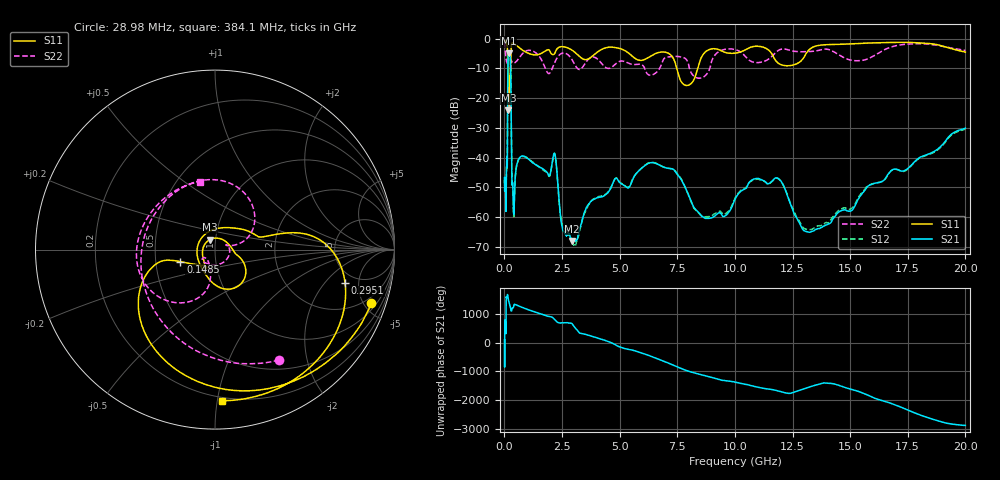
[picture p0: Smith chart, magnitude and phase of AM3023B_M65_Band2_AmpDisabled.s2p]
!Agilent Technologies,E8364B,MY43040894,A.07.50.67
!Agilent E8364B: A.07.50.67
!Date: Tuesday, October 27, 2020 10:48:38
!Correction: S11(Full 2 Port(1,2))
!S21(Full 2 Port(1,2))
!S12(Full 2 Port(1,2))
!S22(Full 2 Port(1,2))
!S2P File: Measurements: S11, S21, S12, S22:Log Frequency Sweep
# Hz S  dB  R 50
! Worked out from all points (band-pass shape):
!   3201 points, 10 MHz to 20 GHz, reference 50 ohm
!   highest |S21| = -4.86 dB at 193.4 MHz (marker M1); lowest = -68.0 dB at 2.92 GHz (marker M2)
!   |S21| within 3 dB of the highest: 154.6 MHz to 264.8 MHz (110.2 MHz wide, 52.6 % of centre)
!   lowest |S11| = -24.1 dB at 175.4 MHz (marker M3), VSWR 1.13, Z = 46.9 + j5.22 ohm
!   |S11| at or under -10 dB: 145.6 MHz to 264.5 MHz (118.9 MHz wide, 58 % of centre); 7.479 GHz to 8.387 GHz (907.2 MHz wide, 11.4 % of centre)
!   |S22| runs from -23.7 to -1.3 dB; largest |S21 - S12| = 0.0085
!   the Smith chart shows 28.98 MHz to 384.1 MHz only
!   S11 on the Smith chart (normalised r, x): 28.98 MHz: 1.43, -5.64; 148.5 MHz: 0.67, -0.09; 295.1 MHz: 3.96, -3.39; 384.1 MHz: 0.18, -1.03
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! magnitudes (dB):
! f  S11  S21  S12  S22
! 10 MHz  -0.6  -47.6  -47.6  -1.3
! 28.98 MHz  -0.7  -49.0  -48.9  -3.0
! 35.55 MHz  -0.8  -48.7  -48.4  -3.6
! 69.3 MHz  -1.1  -57.6  -56.0  -6.4
! 126.1 MHz  -3.0  -41.9  -42.3  -8.2
! 148.5 MHz  -13.8  -11.9  -11.9  -10.4
! 175.4 MHz  -24.1  -5.2  -5.3  -22.3
! 193.4 MHz  -13.5  -4.9  -4.9  -21.4
! 260.2 MHz  -10.9  -6.9  -6.9  -18.8
! 295.1 MHz  -2.5  -25.4  -25.4  -7.1
! 325.3 MHz  -1.5  -47.2  -47.0  -7.7
! 384.1 MHz  -1.5  -54.7  -55.6  -8.2
! 447.2 MHz  -1.8  -50.0  -50.1  -8.1
! 1.59 GHz  -5.0  -43.4  -43.6  -6.8
! 2.181 GHz  -5.0  -38.6  -38.6  -8.0
! 2.92 GHz  -3.8  -68.0  -68.8  -6.9
! 5.639 GHz  -6.4  -46.2  -46.1  -8.7
! 7.939 GHz  -15.7  -51.7  -51.6  -7.5
! 8.834 GHz  -3.8  -60.4  -59.8  -11.3
! 11.64 GHz  -5.5  -47.7  -47.8  -5.7
! 13.42 GHz  -2.7  -64.6  -63.7  -4.2
! 20 GHz  -4.5  -30.1  -30.4  -3.9
